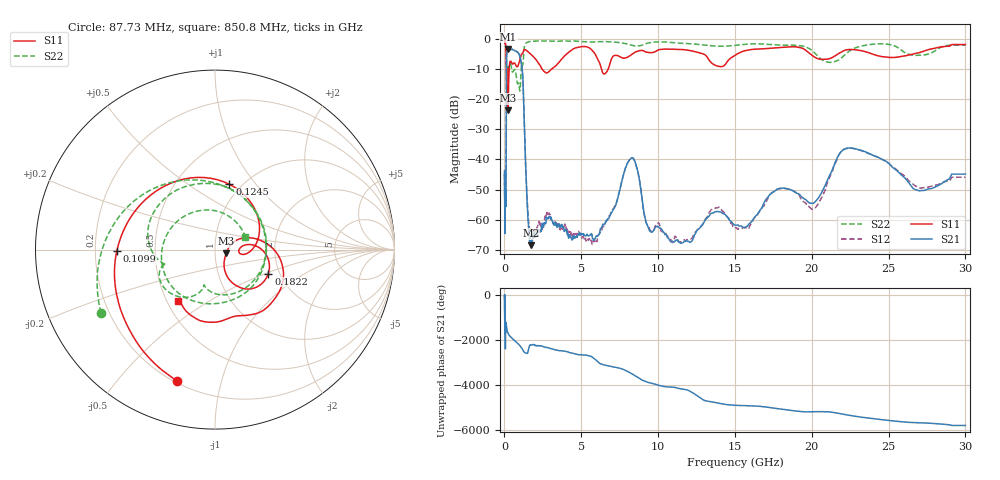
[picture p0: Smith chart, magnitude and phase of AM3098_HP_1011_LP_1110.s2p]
! Date/Time: Thu, Feb 28, 2019 8:43 AM
! Network Analyzer: Agilent Technologies E8364B Rev: A.07.50.67
! Sweep from 0.010 to 30.000 GHz, 1601 Points, Sweep Type: LOG
! Power Supply: 5.022 V, 0.002 A
# Hz S DB R 50
!freq MagS11 AngS11 MagS21 AngS21 MagS12 AngS12 MagS22 AngS22
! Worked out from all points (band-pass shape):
!   1601 points, 10 MHz to 30 GHz, reference 50 ohm
!   highest |S21| = -3.16 dB at 258.6 MHz (marker M1); lowest = -68.5 dB at 1.714 GHz (marker M2)
!   |S21| within 3 dB of the highest: 137.5 MHz to 1.029 GHz (891.1 MHz wide, 153 % of centre)
!   lowest |S11| = -23.6 dB at 242.3 MHz (marker M3), VSWR 1.14, Z = 56.6 - j2.42 ohm
!   |S11| at or under -10 dB: 192.8 MHz to 302.9 MHz (110.1 MHz wide, 44.4 % of centre); 2.471 GHz to 3.037 GHz (565.7 MHz wide, 20.5 % of centre); 6.319 GHz to 6.74 GHz (420.7 MHz wide, 6.44 % of centre)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
!   |S22| runs from -17.2 to -0.5 dB; largest |S21 - S12| = 0.011
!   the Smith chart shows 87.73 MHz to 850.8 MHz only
!   S11 on the Smith chart (normalised r, x): 87.73 MHz: 0.21, -0.73; 109.9 MHz: 0.29, -0.01; 124.5 MHz: 0.88, +0.74; 182.2 MHz: 1.75, -0.52; 850.8 MHz: 0.57, -0.37
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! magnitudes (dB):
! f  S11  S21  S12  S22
! 10 MHz  -0.4  -45.0  -44.7  -0.6
! 38.04 MHz  -0.4  -61.3  -58.8  -0.9
! 87.73 MHz  -2.4  -52.7  -53.8  -2.8
! 97.46 MHz  -3.4  -53.9  -54.2  -3.9
! 109.9 MHz  -5.2  -33.2  -33.0  -6.6
! 124.5 MHz  -8.6  -13.0  -12.9  -10.9
! 144.7 MHz  -17.3  -5.1  -5.1  -13.8
! 182.2 MHz  -9.7  -3.9  -3.8  -9.1
! 242.3 MHz  -23.6  -3.2  -3.1  -10.9
! 258.6 MHz  -18.5  -3.2  -3.1  -10.5
! 550.5 MHz  -8.1  -3.5  -3.4  -10.8
! 850.8 MHz  -9.0  -4.2  -4.2  -14.7
! 1.172 GHz  -4.8  -10.9  -10.8  -8.7
! 1.49 GHz  -3.9  -55.4  -54.3  -0.9
! 1.714 GHz  -4.9  -68.5  -67.1  -0.6
! 2.084 GHz  -6.9  -65.0  -63.5  -0.5
! 5.841 GHz  -4.4  -67.0  -67.5  -0.8
! 7.926 GHz  -6.1  -42.2  -42.1  -1.5
! 11.25 GHz  -3.3  -66.8  -66.1  -1.2
! 20.1 GHz  -5.6  -54.6  -56.5  -4.1
! 22.67 GHz  -3.4  -36.3  -36.3  -3.2
! 30 GHz  -1.7  -44.9  -45.9  -1.9
